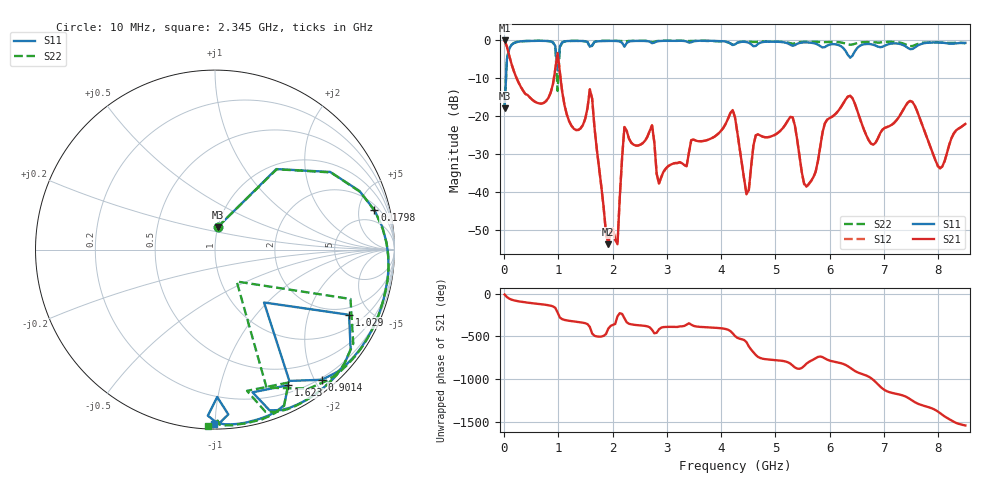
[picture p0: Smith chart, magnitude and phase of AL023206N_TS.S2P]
!AVX CORPORATION
!PN: AL023206N_TS
!DESCRIPTION: AIR CORE INDUCTOR, 206nH, 13 turns
!Agilent Technologies,E5071C,MY46102230,A.09.54
!Date: Mon Sep 03 16:46:03 2012
!Data & Calibration Information:
!Freq	S11:SOLT2(ON)	S21:SOLT2(ON)	S12:SOLT2(ON)	S22:SOLT2(ON)
# Hz S dB R 50
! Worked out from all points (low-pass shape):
!   201 points, 10 MHz to 8.5 GHz, reference 50 ohm
!   highest |S21| = -0.06 dB at 10 MHz (marker M1); lowest = -53.7 dB at 1.92 GHz (marker M2)
!   |S21| within 3 dB of the highest: start of sweep to 77 MHz
!   lowest |S11| = -17.9 dB at 10 MHz (marker M3), VSWR 1.29, Z = 50 + j12.9 ohm
!   |S11| at or under -10 dB: start of sweep to 35.9 MHz
!   |S22| runs from -17.8 to -0.1 dB; largest |S21 - S12| = 0.0065
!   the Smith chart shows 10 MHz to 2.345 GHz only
!   S11 on the Smith chart (normalised r, x): 10 MHz: 1.00, +0.26; 179.8 MHz: 2.68, +7.24; 901.5 MHz: 0.17, -2.10; 1.029 GHz: 1.58, -3.71; 1.623 GHz: 0.29, -1.64; 2.345 GHz: 0.03, -0.99
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1e7  -17.86 82.5  -0.06 -7.9  -0.10 -8.2  -17.81 82.8
1.798e8  -0.77 13.9  -8.12 -76.0  -8.10 -76.0  -0.75 13.4
9.0145e8  -0.55 -50.6  -11.49 -147.0  -11.48 -147.1  -0.60 -56.1
9.8635e8  -7.92 -47.2  -3.37 140.9  -3.36 140.8  -13.35 -55.8
1.0288e9  -1.61 -25.9  -8.37 82.2  -8.37 82.1  -1.90 -20.0
1.4533e9  -0.22 -64.6  -22.29 21.6  -22.28 21.7  -0.21 -65.7
1.6231e9  -1.32 -61.6  -15.38 -105.4  -15.38 -105.4  -1.45 -61.0
1.92025e9  -0.18 -79.5  -53.71 -47.7  -54.17 -50.1  -0.14 -79.6
2.09005e9  -0.23 -87.0  -53.67 96.6  -53.50 92.7  -0.16 -85.5
2.2174e9  -1.71 -89.1  -22.84 76.4  -22.83 76.3  -0.42 -89.2
2.34475e9  -0.24 -90.4  -26.97 2.1  -26.99 2.2  -0.16 -92.1
2.7268e9  -0.78 -103.5  -22.38 -62.0  -22.40 -61.8  -0.54 -102.3
2.85415e9  -0.22 -103.7  -37.73 -56.0  -37.74 -56.2  -0.17 -103.4
4.255e9  -1.09 -115.3  -20.29 -134.5  -20.29 -134.6  -1.06 -128.9
4.46725e9  -0.48 -121.4  -40.49 153.2  -40.50 153.7  -0.35 -135.2
5.2738e9  -1.19 -135.1  -20.19 -97.8  -20.18 -97.9  -0.78 -153.5
5.6983e9  -0.76 -142.9  -36.04 -50.4  -36.17 -51.1  -0.39 -158.4
6.33505e9  -3.87 -157.4  -14.81 -128.8  -14.83 -128.9  -1.07 -165.5
7.09915e9  -0.98 -155.8  -22.59 -73.3  -22.56 -73.2  -0.40 -166.4
7.52365e9  -2.30 -161.8  -16.23 -172.9  -16.22 -173.0  -1.53 -164.6
8.03305e9  -0.63 -173.0  -33.69 41.0  -33.68 41.0  -0.61 -167.0
8.5e9  -0.70 178.3  -22.02 -104.0  -22.00 -103.9  -0.83 -172.9
